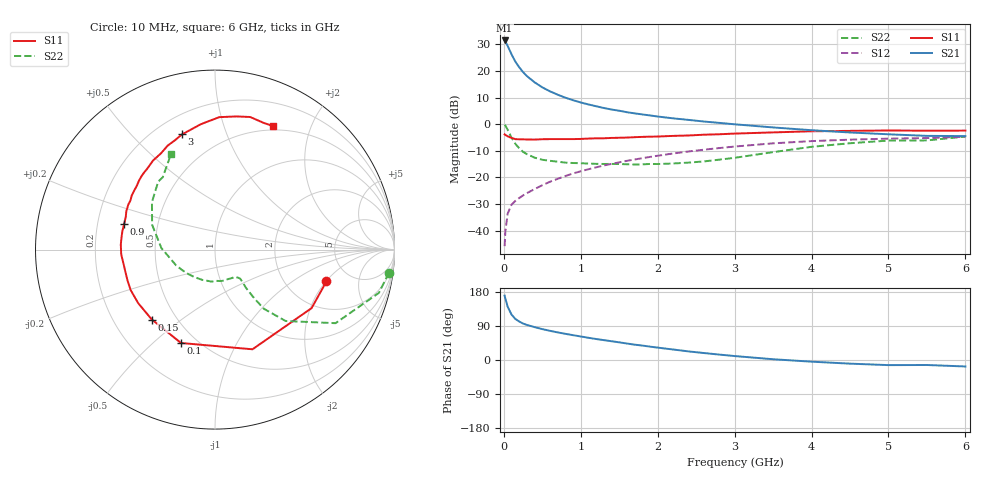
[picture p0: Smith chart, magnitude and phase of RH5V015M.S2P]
! SIEMENS Small Signal Semiconductors
! BFR106
! Si NPN RF Bipolar Junction Transistor in SOT23
! VCE = 5 V  IC = 15 mA
! Common Emitter S-Parameters:  August  1996
# GHz  S  MA  R  50
!  f  S11  S21  S12  S22
! GHz  MAG  ANG  MAG  ANG  MAG  ANG  MAG  ANG
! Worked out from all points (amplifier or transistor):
!   36 points, 10 MHz to 6 GHz, reference 50 ohm
!   highest |S21| = 31.5 dB at 10 MHz (marker M1)
!   |S21| within 3 dB of that: start of sweep to 64.84 MHz
!   unconditionally stable (mu >= 1): 404.7 MHz to 2.091 GHz; 5.468 GHz to 5.674 GHz
!   at 250 MHz: K = 0.82, MSG = 23.2 dB, |S12| = -26.8 dB
!   at 1.4 GHz: K = 1.08, MAG = 8.5 dB, |S12| = -14.9 dB
!   at 6 GHz: K = 1.00, MSG = 0.1 dB, |S12| = -4.7 dB
!   S11 on the Smith chart (normalised r, x): 10 MHz: 3.33, -2.02; 100 MHz: 0.41, -0.62; 150 MHz: 0.37, -0.39; 900 MHz: 0.32, +0.13; 3 GHz: 0.31, +0.71; 6 GHz: 0.45, +1.47
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0.01  0.6459 -15.9  37.67 170.0  0.0051 85.7  0.9774 -7.6
0.02  0.6293 -31.2  36.19 161.8  0.0098 77.7  0.9444 -14.8
0.05  0.5934 -69.4  29.7 140.3  0.0209 63.3  0.7869 -31.4
0.1  0.5538 -110.0  20.66 119.9  0.0307 52.7  0.5598 -45.3
0.15  0.5251 -132.0  15.04 108.2  0.0362 50.9  0.4285 -50.4
0.2  0.5217 -145.1  11.78 101.5  0.041 52.1  0.3537 -51.1
0.25  0.5212 -154.4  9.557 96.2  0.0459 53.8  0.3027 -51.1
0.3  0.5168 -160.8  8.062 92.5  0.0507 55.9  0.2743 -51.0
0.4  0.5155 -170.6  6.149 86.7  0.0605 59.6  0.2354 -49.7
0.5  0.5232 -177.1  4.945 81.5  0.0714 61.9  0.2148 -49.1
0.6  0.5255 177.0  4.161 77.0  0.0831 63.2  0.2056 -50.0
0.7  0.5253 172.2  3.597 72.8  0.0942 64.2  0.1977 -51.7
0.9  0.526 164.1  2.833 65.5  0.119 64.7  0.1867 -55.1
1.1  0.5381 156.7  2.36 58.6  0.1426 64.2  0.1825 -62.0
1.3  0.5449 149.9  2.022 52.4  0.1679 63.1  0.1792 -68.7
1.6  0.5622 140.8  1.685 43.5  0.2052 60.7  0.177 -81.7
2.2  0.6042 124.9  1.292 27.7  0.2822 54.0  0.183 -112.4
3  0.6678 105.9  0.999 10.4  0.381 42.6  0.2341 -158.1
3.5  0.7032 96.4  0.872 2.0  0.4377 34.8  0.2991 178.3
4.5  0.7514 80.9  0.701 -9.6  0.5135 18.3  0.4399 143.0
5.5  0.7562 69.0  0.605 -13.2  0.5501 7.3  0.4973 125.8
6  0.7601 65.0  0.599 -17.1  0.5839 -0.5  0.5863 114.7
